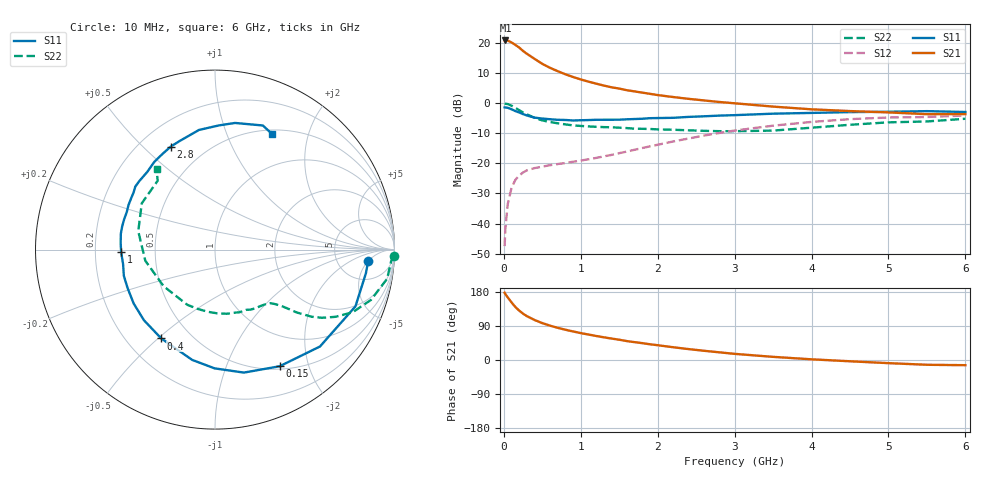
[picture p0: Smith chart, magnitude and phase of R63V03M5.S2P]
! SIEMENS Small Signal Semiconductors
! BFR193
! Si NPN RF Bipolar Junction Transistor in SOT23
! VCE = 3 V  IC = 3.5 mA
! Common Emitter S-Parameters:  May  1996
# GHz  S  MA  R  50
!  f  S11  S21  S12  S22
! GHz  MAG  ANG  MAG  ANG  MAG  ANG  MAG  ANG
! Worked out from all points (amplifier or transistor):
!   36 points, 10 MHz to 6 GHz, reference 50 ohm
!   highest |S21| = 20.9 dB at 20 MHz (marker M1)
!   |S21| within 3 dB of that: start of sweep to 227.8 MHz
!   unconditionally stable (mu >= 1): 994.3 MHz to 2.031 GHz
!   at 250 MHz: K = 0.34, MSG = 20.2 dB, |S12| = -23.0 dB
!   at 1.4 GHz: K = 1.09, MAG = 9.4 dB, |S12| = -17.2 dB
!   at 6 GHz: K = 0.98, MSG = 0.2 dB, |S12| = -4.0 dB
!   S11 on the Smith chart (normalised r, x): 10 MHz: 10, -5; 150 MHz: 0.54, -1.56; 400 MHz: 0.34, -0.51; 1 GHz: 0.31, -0.01; 2.8 GHz: 0.32, +0.61; 6 GHz: 0.55, +1.47
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0.01  0.8557 -4.4  11.08 177.4  0.0042 87.3  0.9962 -1.9
0.02  0.851 -8.9  11.12 174.0  0.0082 86.3  0.9834 -3.8
0.05  0.844 -22.0  11.07 165.4  0.0209 78.0  0.9728 -9.6
0.1  0.796 -42.7  10.31 152.1  0.0391 68.7  0.913 -17.9
0.15  0.7431 -61.0  9.381 139.7  0.0534 60.1  0.8423 -24.5
0.2  0.7039 -76.8  8.454 130.2  0.063 54.3  0.7679 -29.2
0.25  0.6617 -90.2  7.439 122.2  0.0708 49.7  0.7053 -32.6
0.3  0.6275 -101.7  6.668 115.7  0.0767 46.6  0.6554 -34.8
0.4  0.5784 -121.2  5.49 105.5  0.0836 42.8  0.5734 -37.6
0.5  0.5582 -135.2  4.536 97.3  0.0884 41.7  0.5195 -39.1
0.6  0.5436 -146.5  3.899 90.7  0.0934 41.5  0.4885 -40.2
0.8  0.5285 -163.9  3.045 79.9  0.1016 43.8  0.446 -42.6
1  0.523 -178.3  2.496 71.0  0.1116 48.0  0.4205 -45.7
1.1  0.5268 176.2  2.296 67.2  0.1171 50.0  0.4126 -47.8
1.3  0.5331 166.0  1.975 59.9  0.1311 53.4  0.402 -51.9
1.6  0.5421 152.7  1.652 49.9  0.1577 57.5  0.3873 -59.8
2.2  0.5741 131.2  1.273 33.7  0.2316 59.0  0.3635 -79.5
2.8  0.6247 113.2  1.053 20.3  0.321 53.7  0.3441 -106.3
3.5  0.6727 97.6  0.882 8.3  0.4247 42.4  0.3516 -144.5
4.5  0.7145 81.0  0.743 -3.4  0.5451 24.3  0.4397 166.5
5.5  0.7412 68.9  0.66 -12.6  0.592 6.2  0.4992 129.8
6  0.7177 63.6  0.662 -13.7  0.6274 1.1  0.5537 126.0
